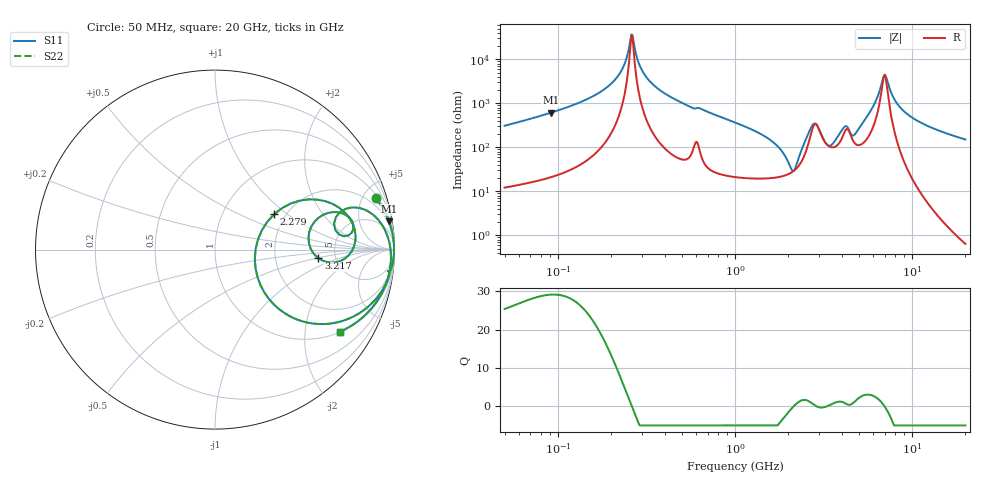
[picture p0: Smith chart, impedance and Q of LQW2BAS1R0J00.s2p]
!Murata Part Number: LQW2BAS1R0J00
!These Parameters are Measured in Series Mode Connection
!  o--[Z]--o
!Port1  Port2
!  o-------o
!Freq. Start=50[MHz] Stop=20[GHz], 401[Steps]
# Hz S RI R 50
!Freq.(Hz) S11(Real) S11(Imag) S21(Real) S21(Imag) S12(Real) S12(Imag) S22(Real) S22(Imag)
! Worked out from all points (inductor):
!   401 points, 50 MHz to 20 GHz, reference 50 ohm
!   read as one part in series: L = 944 nH near 51.52 MHz
!   highest Q = 29.1 at 91.03 MHz (marker M1), where L = 1.07 uH
!   self-resonance near 259.7 MHz
!   S11 on the Smith chart (normalised r, x): 50 MHz: 1.24, +6.19; 2.279 GHz: 1.74, +0.80; 3.217 GHz: 3.65, -0.53; 20 GHz: 1.01, -3.02
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5e7  0.8964 0.2857  0.1036 -0.2857  0.1036 -0.2857  0.8964 0.2857
9.102821e7  0.9688 0.1576  0.0312 -0.1576  0.0312 -0.1576  0.9688 0.1576
1.364002e8  0.9884 0.0896  0.0116 -0.0896  0.0116 -0.0896  0.9884 0.0896
2.137812e8  0.9967 0.0265  0.00332 -0.0265  0.00332 -0.0265  0.9967 0.0265
2.374136e8  0.9973 0.0127  0.00273 -0.0127  0.00273 -0.0127  0.9973 0.0127
2.597386e8  0.9974 0.000879  0.00258 -0.000879  0.00258 -0.000879  0.9974 0.000879
3.017088e8  0.997 -0.0189  0.00305 0.0189  0.00305 0.0189  0.997 -0.0189
3.721004e8  0.9946 -0.0479  0.0054 0.0479  0.0054 0.0479  0.9946 -0.0479
1e9  0.919 -0.2456  0.081 0.2456  0.081 0.2456  0.919 -0.2456
1.766834e9  0.4995 -0.4031  0.5005 0.4031  0.5005 0.4031  0.4995 -0.4031
2.114743e9  0.2219 -0.0512  0.7781 0.0512  0.7781 0.0512  0.2219 -0.0512
2.279204e9  0.3287 0.1962  0.6713 -0.1962  0.6713 -0.1962  0.3287 0.1962
2.728004e9  0.777 0.1162  0.223 -0.1162  0.223 -0.1162  0.777 0.1162
3.216634e9  0.5758 -0.0481  0.4242 0.0481  0.4242 0.0481  0.5758 -0.0481
3.736399e9  0.6311 0.2048  0.3689 -0.2048  0.3689 -0.2048  0.6311 0.2048
4.212059e9  0.7714 0.1167  0.2286 -0.1167  0.2286 -0.1167  0.7714 0.1167
4.81993e9  0.7247 0.2256  0.2753 -0.2256  0.2753 -0.2256  0.7247 0.2256
6.034176e9  0.9511 0.0999  0.0489 -0.0999  0.0489 -0.0999  0.9511 0.0999
6.905011e9  0.9771 0.00731  0.0229 -0.00731  0.0229 -0.00731  0.9771 0.00731
7.442007e9  0.9804 -0.0388  0.0196 0.0388  0.0196 0.0388  0.9804 -0.0388
1.004137e10  0.9494 -0.1999  0.0506 0.1999  0.0506 0.1999  0.9494 -0.1999
2e10  0.6939 -0.4588  0.3061 0.4588  0.3061 0.4588  0.6939 -0.4588
